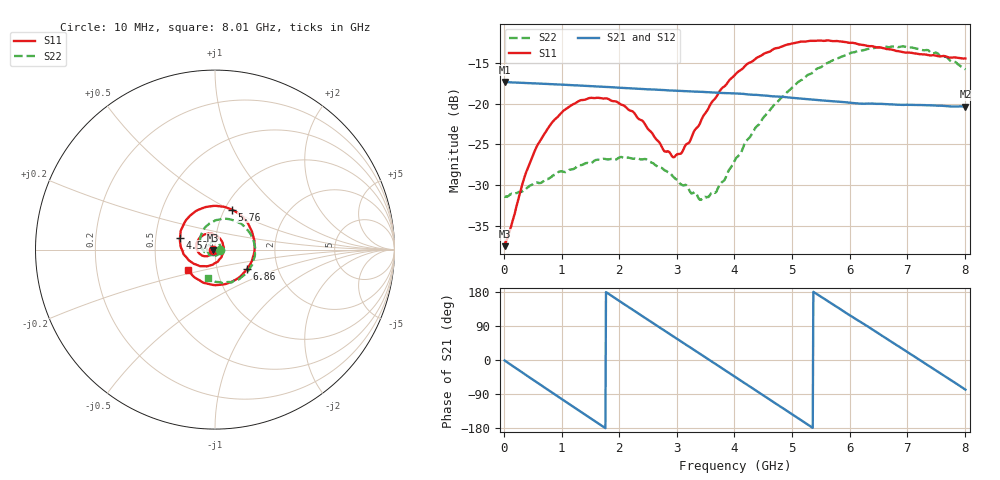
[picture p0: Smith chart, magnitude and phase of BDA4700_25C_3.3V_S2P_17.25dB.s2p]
!Agilent Technologies,E5071B,MY42404982,A.09.10
!Date: Mon Oct 20 18:10:17 2025
!Data & Calibration Information:
!Freq	S11:SOLT2(ON)	S21:SOLT2(ON)	S12:SOLT2(ON)	S22:SOLT2(ON)
# Hz S RI R 50
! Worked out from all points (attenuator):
!   801 points, 10 MHz to 8.01 GHz, reference 50 ohm
!   highest |S21| = -17.34 dB at 10 MHz (marker M1); lowest = -20.4 dB at 8.01 GHz (marker M2)
!   lowest |S11| = -37.5 dB at 10 MHz (marker M3), VSWR 1.03, Z = 48.7 - j0.142 ohm
!   |S11| at or under -10 dB: start of sweep to end of sweep
!   |S22| runs from -31.8 to -13.0 dB; largest |S21 - S12| = 0.0016
!   S11 on the Smith chart (normalised r, x): 10 MHz: 0.97, -0.00; 4.57 GHz: 0.67, +0.09; 5.76 GHz: 1.09, +0.51; 6.86 GHz: 1.40, -0.31; 8.01 GHz: 0.72, -0.17
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1e7  -0.0132 -0.00145  0.1358 -0.00294  0.1357 -0.00308  0.0268 -0.000876
3.6e8  -0.0242 -0.0263  0.1061 -0.0814  0.1061 -0.0814  0.0224 -0.019
5.8e8  -0.0417 -0.0365  0.0663 -0.1149  0.0664 -0.1149  0.0142 -0.0294
8.7e8  -0.0715 -0.0333  0.000916 -0.1312  0.000934 -0.1313  -0.00699 -0.0358
1.35e9  -0.1041 0.0143  -0.0963 -0.0855  -0.0962 -0.0856  -0.0381 -0.0173
1.77e9  -0.0822 0.0694  -0.1264 0.0018  -0.1265 0.00185  -0.0429 0.0153
2.07e9  -0.0409 0.0884  -0.1068 0.0643  -0.107 0.0642  -0.0291 0.0363
2.68e9  0.0409 0.0419  0.00415 0.1213  0.00394 0.1212  0.017 0.037
2.97e9  0.0464 -0.00999  0.0613 0.103  0.0611 0.1028  0.029 0.0187
3.09e9  0.0396 -0.0308  0.0812 0.0875  0.0804 0.0879  0.0304 0.00858
3.42e9  -0.00444 -0.0782  0.1142 0.0297  0.1143 0.0296  0.0196 -0.0164
3.68e9  -0.058 -0.0923  0.1143 -0.0228  0.1144 -0.0233  -4.6e-05 -0.0285
4.01e9  -0.1333 -0.0687  0.0825 -0.0805  0.0826 -0.0803  -0.0353 -0.0276
4.57e9  -0.1954 0.0647  -0.0203 -0.1097  -0.02 -0.1098  -0.081 0.0315
4.94e9  -0.1561 0.1706  -0.0801 -0.0739  -0.0799 -0.0744  -0.0727 0.0949
5.35e9  -0.0427 0.2386  -0.1058 -0.00372  -0.1058 -0.00446  -0.014 0.1534
5.76e9  0.0957 0.2224  -0.0809 0.0635  -0.0808 0.0636  0.0798 0.1694
6.23e9  0.2041 0.1038  -0.0115 0.0989  -0.0101 0.0992  0.1837 0.1062
6.68e9  0.2089 -0.0518  0.0601 0.0785  0.0604 0.0784  0.2217 -0.00873
6.86e9  0.1792 -0.1079  0.0804 0.0565  0.0807 0.0559  0.214 -0.0598
7.45e9  0.00278 -0.1982  0.0896 -0.0378  0.0897 -0.0379  0.104 -0.1744
8.01e9  -0.1529 -0.1116  0.0196 -0.0937  0.0199 -0.0938  -0.038 -0.1573
